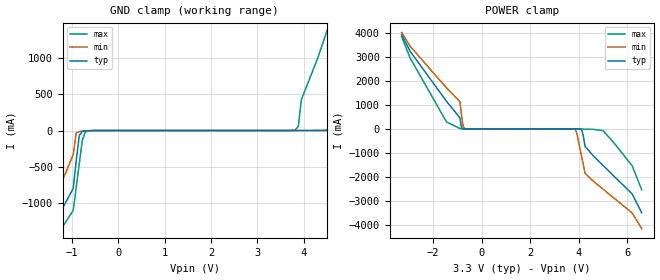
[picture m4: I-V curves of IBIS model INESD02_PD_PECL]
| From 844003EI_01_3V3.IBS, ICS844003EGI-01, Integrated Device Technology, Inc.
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[Model]   INESD02_PD_PECL
Model_type  Input
Polarity   Non-Inverting
Vinl = 0.8V
Vinh = 2.0V
|   typ   min   max
C_comp   2pF   1.5pF   2.5pF
|   typ   min   max
[Voltage range]  3.3V   3.135V   3.465V
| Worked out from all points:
|   GND clamp passes 1 mA (typ) near -0.59 V on its own axis
|   POWER clamp passes 1 mA (typ) near -0.70 V on its own axis
[GND_clamp]
-3.3V     -3.894A    -4.294A    -3.674A
-1.6V     -1.569A    -1.322A    -1.74A
-974.8mV  -794.1mA   -331.5mA   -1.096A
-843.4mV  -68.33mA   -15.34mA   -452.9mA
-646.5mV  -1.912mA   -4.151mA   -2.665mA
3.818V    89.38uA    70.49uA    7.198mA
3.95V     342.2uA    75.94uA    423.8mA
4.6V      7.437mA    165.5uA    1.553A
4.9V      78.32mA    440.9uA    2.118A
5.5V      1.293A     2.769mA    3.249A
6.25V     2.651A     112.4mA    4.38A
6.6V      3.331A     896.1mA    4.946A
[POWER_clamp]
-3.3V     3.923A     4.017A     3.838A
-2.95V    3.23A      3.44A      2.951A
-1.45V    1.149A     1.709A     289.6mA
-896.9mV  456.5mA    1.133A     15.4mA
-762.9mV  4.223mA    91.07mA    1.486mA
-695.9mV  792.2uA    10.73mA    555.6uA
3.861V    -556.7uA   -26.14mA   -39.45uA
4.129V    -41.85mA   -1.19A     -4.904mA
4.263V    -724.2mA   -1.847A    -12.04mA
5V        -1.514A    -2.505A    -71.38mA
6.2V      -2.701A    -3.492A    -1.525A
6.6V      -3.492A    -4.151A    -2.536A
